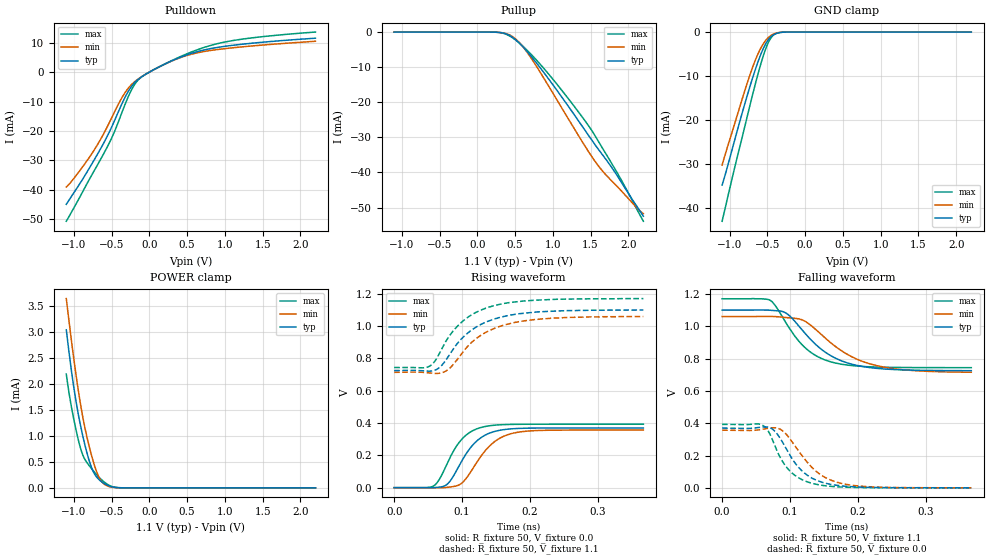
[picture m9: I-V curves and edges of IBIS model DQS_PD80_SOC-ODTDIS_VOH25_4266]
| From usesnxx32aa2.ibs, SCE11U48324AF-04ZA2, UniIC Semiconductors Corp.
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| DQS_PD80_SOC-ODTDIS_VOH25_4266
| (80 Ohm Pulldown, SOC ODT disabled setting, VOH=VDDQ/2.5 cal. point, 3200-4266Mbps)
[Model]   DQS_PD80_SOC-ODTDIS_VOH25_4266
Model_type   I/O
Vinl = 160.000mV
Vinh = 280.000mV
Vmeas = 220.000mV
Vref = 0.0mV
Cref = 0.0pF
|   typ   min   max
|C_comp   0.838pF   0.788pF   0.888pF
C_comp_pullup   0.4190pF   0.3940pF   0.4440pF
C_comp_pulldown   0.4190pF   0.3940pF   0.4440pF
| Note: C_comp changes when the ODT circuit is enabled.
[Model Spec]
| Input threshold voltage corners
Vinl   0.1600V   0.1520V   0.1740V
Vinh   0.2800V   0.2720V   0.2940V
| Measurement voltage corners
Vmeas   0.2200V   0.2120V   0.2340V
| Timing spec test load voltage corners
Vref   0.0000V   0.0000V   0.0000V
| Dynamic Overshoot Parameters from LPDDR4 Specification
D_overshoot_ampl_h   0.30   NA   NA
D_overshoot_ampl_l   0.30   NA   NA
D_overshoot_area_h   0.1n   NA   NA
D_overshoot_area_l   0.1n   NA   NA
[Receiver Thresholds]
Vcross_low   = 160.0mV
Vcross_high  = 280.0mV
Vdiff_ac   = 120mV
Vdiff_dc   = 120mV
Tdiffslew_ac = 10.000ns |Not specified, so set to high value
[Voltage Range]   1.1000V   1.0600V   1.1700V
[Pullup Reference]   1.1000V   1.0600V   1.1700V
| Junction Temperature (Ambient temp is 35C typ 95C min -40C max)
[Temperature Range]   50.0   110.0   -40.0
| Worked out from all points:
|   slope of the pulldown table from 0 to 0.165 V, typ, clamps not added: 73.8 ohm
|   slope of the pullup table from 0 to 0.165 V, typ, clamps not added: 17.5 kohm
|   GND clamp passes 1 mA (typ) near -0.45 V on its own axis
|   POWER clamp passes 1 mA (typ) near -0.88 V on its own axis
|   rising waveform, R_fixture 50, V_fixture 0.0: 20-80 % time 35.9ps typ, 39.5ps min, 32.8ps max; typ from 0.001 V to 0.37 V
|   falling waveform, R_fixture 50, V_fixture 1.1: 20-80 % time 59.9ps typ, 70.7ps min, 48.8ps max; typ from 1.1 V to 0.725 V
|   rising waveform, R_fixture 50, V_fixture 1.1: 20-80 % time 57.7ps typ, 59.1ps min, 54.1ps max; typ from 0.725 V to 1.1 V
|   falling waveform, R_fixture 50, V_fixture 0.0: 20-80 % time 39.7ps typ, 45.7ps min, 34.3ps max; typ from 0.37 V to 0.001 V
[Pulldown]
|   Voltage   I(typ)   I(min)   I(max)
-1.1V     -44.88mA   -39.02mA   -50.64mA
-948.2mV  -38.97mA   -34.38mA   -43.73mA
-723.8mV  -29.53mA   -26.19mA   -33.19mA
-611.6mV  -24.44mA   -21.26mA   -28.03mA
-496.1mV  -18.51mA   -15.39mA   -22.23mA
-317.9mV  -8.375mA   -6.836mA   -10.74mA
-215.6mV  -4.219mA   -3.747mA   -5.086mA
-110mV    -1.768mA   -1.706mA   -1.813mA
385mV     4.755mA    4.648mA    4.931mA
840.4mV   8.088mA    7.426mA    9.228mA
1.375V    9.824mA    8.884mA    11.65mA
2.2V      11.49mA    10.45mA    13.57mA
[GND Clamp]
|   Voltage   I(typ)   I(min)   I(max)
-1.1V     -34.89mA   -30.35mA   -43.14mA
-941.6mV  -25.14mA   -21.33mA   -31.48mA
-793.1mV  -15.99mA   -13.01mA   -21.07mA
-720.5mV  -11.8mA    -9.215mA   -15.96mA
-661.1mV  -8.6mA     -6.453mA   -11.91mA
-588.5mV  -5.13mA    -3.689mA   -7.336mA
-519.2mV  -2.579mA   -1.835mA   -3.674mA
-466.4mV  -1.302mA   -943.2uA   -1.695mA
-410.3mV  -533.8uA   -393.2uA   -578.9uA
-344.3mV  -144.4uA   -109.5uA   -124uA
-242mV    -10.13uA   -9.161uA   -5.671uA
2.2V      0A         0A         0A
[Pullup]
|   Voltage   I(typ)   I(min)   I(max)
-1.1V     4.112uA    7.441uA    1.363uA
259.6mV   -60.48uA   -59.43uA   -61.39uA
394.9mV   -632.8uA   -526.4uA   -751uA
510.4mV   -2.22mA    -2.012mA   -2.306mA
619.3mV   -4.537mA   -4.575mA   -4.333mA
748mV     -7.82mA    -8.539mA   -7.138mA
1.032V    -15.9mA    -18.5mA    -14.23mA
1.441V    -28.41mA   -32.96mA   -25.69mA
1.589V    -32.98mA   -37.7mA    -30.6mA
1.688V    -35.82mA   -40.32mA   -34.15mA
1.91V     -42.82mA   -45.28mA   -42.24mA
2.2V      -52.46mA   -51.74mA   -53.91mA
[POWER Clamp]
|   Voltage   I(typ)   I(min)   I(max)
-1.1V     3.036mA    3.636mA    2.186mA
-1.044V   2.383mA    2.969mA    1.654mA
-984.5mV  1.784mA    2.311mA    1.206mA
-915.2mV  1.225mA    1.641mA    781.2uA
-852.5mV  818.6uA    1.149mA    543.8uA
-773.3mV  420.9uA    665.5uA    384.1uA
-710.6mV  232.4uA    359.1uA    273.1uA
-654.5mV  142.7uA    170.4uA    185.9uA
-598.4mV  83.65uA    71.96uA    113.1uA
-489.5mV  17.84uA    10.83uA    22.44uA
-374mV    1.397uA    995nA      1.126uA
2.2V      0A         0A         0A
[Ramp]
|   typ   min   max
| 20% - 80%
dV/dt_r   221.42m/35.92p   213.80m/39.54p   235.53m/32.81p
dV/dt_f   224.81m/59.82p   206.68m/70.70p   255.68m/48.88p
| 25% - 75%
|dV/dt_r   184.52m/28.60p   178.17m/31.53p   196.27m/26.12p
|dV/dt_f   187.34m/47.52p   172.23m/56.29p   213.07m/38.85p
R_load = 50
[Rising Waveform]
R_fixture = 50
V_fixture = 0.0
|   Time   V(typ)   V(min)   V(max)
0s        839.9uV    689.3uV    615.3uV
56ps      493.7uV    -4.218uV   7.127mV
65ps      3.273mV    -430.5uV   42.08mV
76ps      15.49mV    1.724mV    131.9mV
101ps     176.3mV    34.14mV    306.8mV
115ps     261mV      113.3mV    351.6mV
130ps     316mV      207.7mV    375.3mV
154ps     354.4mV    302.8mV    389mV
184ps     367.2mV    344.7mV    392.6mV
367ps     369.9mV    357mV      393.2mV
[Falling Waveform]
R_fixture   = 50
V_fixture   = 1.1
V_fixture_min = 1.06
V_fixture_max = 1.17
|   Time   V(typ)   V(min)   V(max)
0s        1.1V       1.06V      1.17V
71ps      1.099V     1.061V     1.16V
79ps      1.096V     1.06V      1.124V
94ps      1.082V     1.054V     1.022V
119ps     971.7mV    1.037V     880.3mV
138ps     886.8mV    979.5mV    818.4mV
162ps     813.2mV    891mV      777.7mV
197ps     759.3mV    799.2mV    754.4mV
236ps     736.5mV    748.9mV    746.6mV
367ps     725.3mV    715.5mV    743.9mV
[Rising Waveform]
R_fixture   = 50
V_fixture   = 1.1
V_fixture_min = 1.06
V_fixture_max = 1.17
|   Time   V(typ)   V(min)   V(max)
0s        724.9mV    713.8mV    743.8mV
51ps      721mV      710.4mV    749.8mV
60ps      727.1mV    707.3mV    783.7mV
73ps      771.8mV    715.4mV    883.4mV
88ps      864.9mV    767.5mV    975.8mV
105ps     945.2mV    859.4mV    1.044V
122ps     997.1mV    926.6mV    1.088V
143ps     1.037V     977.8mV    1.122V
219ps     1.089V     1.045V     1.163V
367ps     1.1V       1.059V     1.17V
[Falling Waveform]
R_fixture = 50
V_fixture = 0.0
|   Time   V(typ)   V(min)   V(max)
0s        370mV      357.1mV    393.3mV
56ps      375.6mV    360.3mV    393.6mV
72ps      369.1mV    371.5mV    319.1mV
85ps      310.3mV    364.2mV    192.9mV
97ps      223.8mV    319.4mV    117.8mV
114ps     120.8mV    220.6mV    59.35mV
133ps     59.32mV    123.8mV    27.9mV
157ps     24.53mV    53.78mV    11.03mV
191ps     7.487mV    16.71mV    3.339mV
367ps     900.1uV    812.3uV    640.9uV
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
